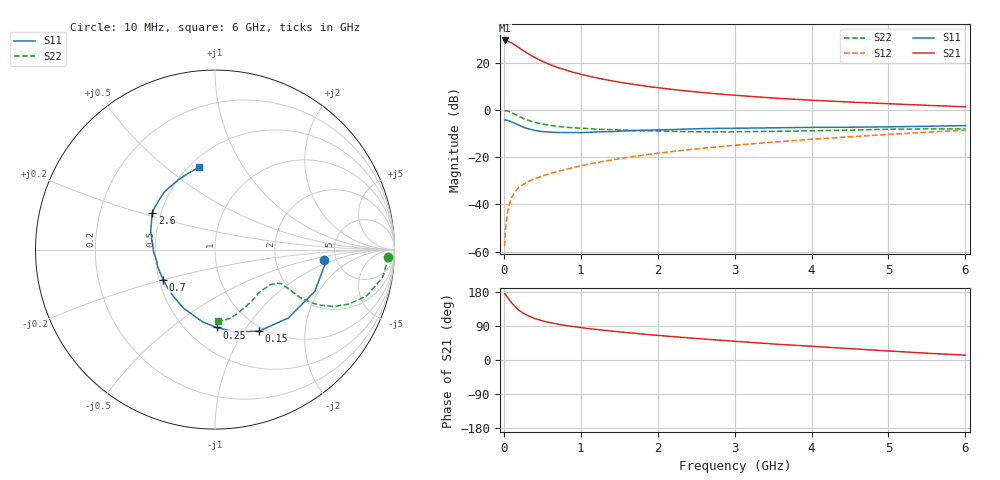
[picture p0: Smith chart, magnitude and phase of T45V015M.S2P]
! Infineon Technologies  Discrete & RF Semiconductors
! BFR182T
! Si NPN RF Bipolar Junction Transistor in SC75
! VCE = 5 V  IC = 15 mA
! Common Emitter S-Parameters:  October  1999
# GHz  S  MA  R  50
!  f  S11  S21  S12  S22
! GHz  MAG  ANG  MAG  ANG  MAG  ANG  MAG  ANG
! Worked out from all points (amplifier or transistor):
!   36 points, 10 MHz to 6 GHz, reference 50 ohm
!   highest |S21| = 29.5 dB at 10 MHz (marker M1)
!   |S21| within 3 dB of that: start of sweep to 193.1 MHz
!   unconditionally stable (mu >= 1): 829.8 MHz to 3.731 GHz
!   at 250 MHz: K = 0.55, MSG = 28.4 dB, |S12| = -31.6 dB
!   at 1.4 GHz: K = 1.08, MAG = 15.0 dB, |S12| = -21.2 dB
!   at 6 GHz: K = 0.85, MSG = 4.9 dB, |S12| = -8.5 dB
!   S11 on the Smith chart (normalised r, x): 10 MHz: 3.97, -0.75; 150 MHz: 0.95, -1.17; 250 MHz: 0.69, -0.74; 700 MHz: 0.53, -0.20; 2.6 GHz: 0.45, +0.22; 6 GHz: 0.56, +0.66
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0.01  0.6097 -5.6  29.76 175.5  0.0013 85.3  0.9646 -2.5
0.02  0.6178 -7.7  29.7 173.7  0.0028 101.6  0.9629 -3.6
0.05  0.603 -22.6  28.89 164.5  0.0073 81.5  0.9475 -9.2
0.1  0.5589 -42.9  26.43 151.1  0.0139 73.8  0.8845 -16.9
0.15  0.5165 -61.5  23.49 139.7  0.019 67.6  0.8027 -22.3
0.2  0.4724 -76.4  20.71 130.8  0.0235 64.7  0.7315 -25.7
0.25  0.4339 -88.8  18.21 123.8  0.0263 62.9  0.6673 -27.7
0.3  0.4075 -100.1  16.12 118.2  0.0297 62.4  0.6199 -28.8
0.4  0.3706 -118.2  12.98 109.5  0.0348 61.7  0.5468 -29.4
0.5  0.3494 -131.0  10.79 103.5  0.0399 62.7  0.5033 -28.7
0.6  0.3386 -141.5  9.157 98.6  0.0449 63.5  0.4717 -28.3
0.7  0.334 -150.0  7.98 94.7  0.05 65.1  0.4489 -27.8
0.9  0.333 -163.8  6.314 88.4  0.0603 66.7  0.4192 -27.5
1.1  0.3364 -174.2  5.231 82.9  0.0712 67.7  0.4027 -28.0
1.3  0.3457 178.2  4.471 78.4  0.0824 68.5  0.3879 -29.0
1.6  0.3611 168.7  3.663 72.3  0.0984 68.9  0.3724 -31.0
2.2  0.3854 156.5  2.717 61.7  0.1322 68.5  0.3528 -37.6
2.6  0.4031 149.8  2.331 55.3  0.1555 67.4  0.3445 -42.5
3.5  0.4184 137.1  1.794 42.3  0.2084 64.2  0.3531 -54.9
4.5  0.431 124.7  1.473 30.0  0.2704 59.3  0.3751 -69.7
5.5  0.4514 108.8  1.256 17.9  0.3382 53.6  0.3964 -82.4
6  0.4672 101.0  1.167 12.8  0.3741 50.0  0.3968 -87.4
